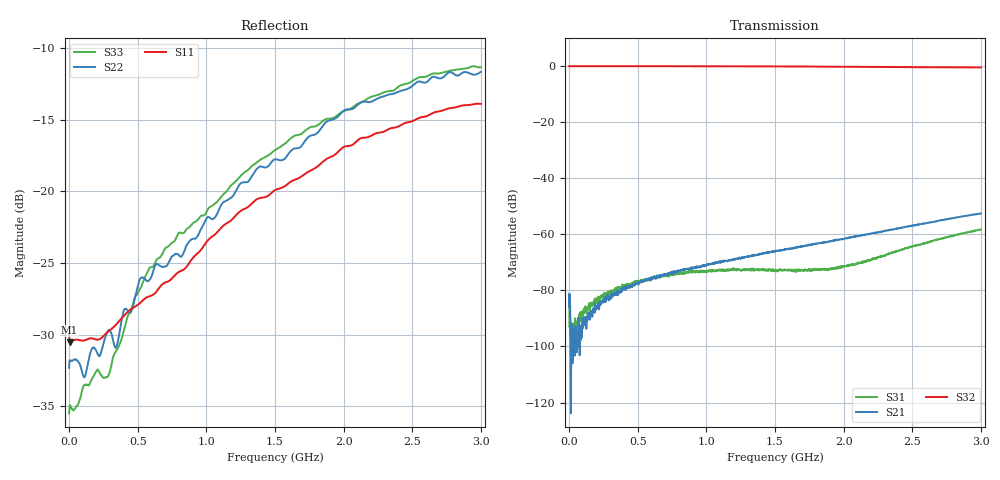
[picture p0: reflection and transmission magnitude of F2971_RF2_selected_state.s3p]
! Frequency:  300kHz to 3GHz
! Package:  4mm x 4mm LQFN Plastic Package: 20 pin with exposed paddle.
!  Pin 1,2,4,5,6,7,9,10,11,12,14,15,18,19 = GND
!  Pin 3  = RF1  = Port 1
!  Pin 8  = RFC  = Port 3
!  Pin 13 = RF2  = Port 2
!  Pin 16 = C2
!  Pin 17 = C1
!  Pin 20 = VDD
!  E.P.  = GND
! State:  RF2 Selected State
! Voltage:  VDD  = +3.0V
!  C1  =  0V (Logic LOW)
!  C2  = +3.0V (Logic HIGH)
! Data:  The device was measured on the F2971 EVKit using a calibrated
!  network analyzer. The results below remove the PCB trace and
!  connector effects using the Automatic Fixture Removal software
!  from Keysight. Therfore, the reference plane for these results
!  are at the device's RF pin.
! Misc:
! Date:  2018-03-27  SJ
! Note:
!  Integrated Device Technology supplies this data as a sample of
!  measured data. Data was taken at 25 degrees C. Integrated Device
!  Technology reserves the right to change this data at anytime.
! Created Tue Mar 27 18:48:21 2018
# hz S db R 75
! 3 Port Network Data from SP1.SP block
! freq  dbS11  angS11  dbS12  angS12  dbS13  angS13
!  dbS21  angS21
!  dbS22  angS22  dbS23  angS23
!  dbS31  angS31  dbS32  angS32
!  dbS33  angS33
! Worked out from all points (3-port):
!   1601 points, 30 kHz to 3 GHz, reference 75 ohm
!   strongest paths, dB at 30 kHz, 750 MHz, 1.5 GHz, 2.25 GHz, 3 GHz:
!     S32: -0.2, -0.2, -0.3, -0.5, -0.7
!     S21: -81.4, -73.6, -66.1, -59.4, -52.7
!     S31: -81.4, -74.3, -72.8, -68.2, -58.4
!   lowest |S11| = -30.5 dB at 3.78 MHz (marker M1), VSWR 1.06, Z = 70.7 + j0.0819 ohm
!   |S11| at or under -10 dB: start of sweep to end of sweep
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30000  -29.95 173.8  -84.72 -17.1  -85.86 69.9
       -81.42 122.2  -32.32 21.7  -0.23 0.1
       -81.45 -61.3  -0.23 0.2  -35.49 44.3
3779962  -30.53 178.9  -91.12 -163.2  -86.84 51.4
         -81.33 144.0  -31.82 0.7  -0.22 -0.1
         -93.20 146.6  -0.22 -0.1  -35.04 4.2
1.125289e8  -30.39 -177.7  -90.45 71.4  -87.65 64.8
            -90.14 86.5  -32.97 -26.3  -0.22 -2.3
            -87.38 62.6  -0.22 -2.3  -33.50 -29.2
2.794022e8  -29.82 -170.4  -82.62 101.7  -81.08 75.0
            -81.66 97.3  -29.78 -51.5  -0.23 -5.7
            -81.47 74.6  -0.22 -5.7  -32.93 -56.8
3.750262e8  -28.94 -164.9  -79.57 99.3  -80.11 75.7
            -80.92 94.7  -29.40 -72.3  -0.23 -7.6
            -78.97 77.9  -0.23 -7.6  -30.51 -73.2
5.775242e8  -27.34 -151.9  -76.30 103.7  -75.87 81.3
            -76.08 100.3  -26.24 -82.9  -0.23 -11.7
            -76.13 82.5  -0.23 -11.7  -25.49 -82.4
8.756462e8  -24.99 -147.2  -72.39 109.3  -73.45 82.2
            -72.32 109.6  -23.49 -101.5  -0.24 -17.7
            -73.28 83.1  -0.24 -17.7  -22.50 -86.8
1.500015e9  -19.92 -136.6  -66.05 127.7  -72.90 103.4
            -66.07 126.5  -17.76 -114.7  -0.30 -30.5
            -72.85 101.5  -0.30 -30.5  -17.11 -105.6
1.955635e9  -17.28 -137.4  -61.97 136.5  -71.97 142.2
            -62.05 135.5  -14.80 -128.0  -0.41 -39.8
            -71.83 141.6  -0.41 -39.8  -14.67 -119.3
3e9  -13.89 -133.1  -52.66 136.3  -58.41 174.6
     -52.68 136.6  -11.66 -144.5  -0.67 -60.0
     -58.35 174.4  -0.66 -60.1  -11.33 -150.4
